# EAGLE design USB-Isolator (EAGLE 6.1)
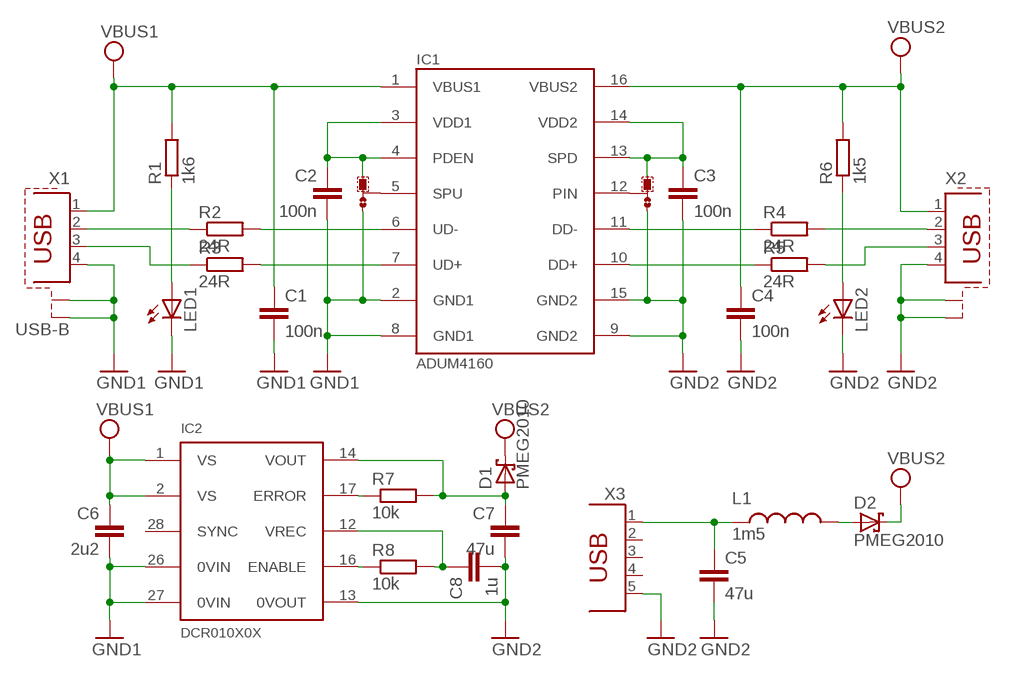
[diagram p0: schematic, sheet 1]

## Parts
C1  100n  C-EUC1206  [C1206]
C2  100n  C-EUC1206  [C1206]
C3  100n  C-EUC1206  [C1206]
C4  100n  C-EUC1206  [C1206]
C5  47u  C-EUC1210  [C1210]
C6  2u2  C-EUC1206  [C1206]
C7  47u  C-EUC1210  [C1210]
C8  1u  C-EUC1206  [C1206]
D1  PMEG2010  [SOD523]
D2  PMEG2010  [SOD523]
IC1  ADUM4160  ADUM4160BRWZ  [SOIC16W]
IC2  DCR010X0X  [SO28-3/12]
JMP1  0R-JUMPA  [A0R-JMP]
JMP2  0R-JUMPA  [A0R-JMP]
L1  1m5  L-1206  [L1206]
LED1  LED3MM  [LED3MM]
LED2  LED3MM  [LED3MM]
R1  1k6  R-EU_M1206  [M1206]
R2  24R  R-EU_M1206  [M1206]
R3  24R  R-EU_M1206  [M1206]
R4  24R  R-EU_M1206  [M1206]
R5  24R  R-EU_M1206  [M1206]
R6  1k5  R-EU_M1206  [M1206]
R7  10k  R-EU_M1206  [M1206]
R8  10k  R-EU_M1206  [M1206]
X1  USB-B  [USB-B]
X2  USB-A-SMD  [USB-A-SMD]
X3  USB-MINI-B-SMD  [USB-MINI-B-SMD]

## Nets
0V: C3.2 C4.2 C5.2 C7.2 C8.2 IC1.9(GND2) IC1.15(GND2) IC2.13(0VOUT) JMP2.3 LED2.K(C) X2.4 X2.P$1(S1) X2.P$2(S2) X3.5 ; supply symbol labelled GND2
GND: C1.2 C2.2 C6.2 IC1.2(GND1) IC1.8(GND1) IC2.26(0VIN) IC2.27(0VIN) JMP1.3 LED1.K(C) X1.4 X1.S1 X1.S2 ; supply symbol labelled GND1
N$1: R2.1 X1.2
N$2: IC1.6(UD-) R2.2
N$3: R3.1 X1.3
N$4: IC1.7(UD+) R3.2
N$5: LED1.A R1.1
N$6: IC1.11(DD-) R4.1
N$7: IC1.10(DD+) R5.1
N$8: R5.2 X2.3
N$9: R4.2 X2.2
N$10: LED2.A R6.1
N$11: IC1.5(SPU) JMP1.2
N$12: IC1.12(PIN) JMP2.2
N$13: C5.1 L1.1 X3.1
N$14: IC2.17(ERROR) R7.1
N$15: IC2.16(ENABLE) R8.1
N$16: C8.1 IC2.12(VREC) R8.2
N$17: D2.A L1.2
N$18: C7.1 D1.A IC2.14(VOUT) R7.2
VBUS1: C1.1 C6.1 IC1.1(VBUS1) IC2.1(VS) IC2.2(VS) R1.2 X1.1
VBUS2: C4.1 D1.C D2.C IC1.16(VBUS2) R6.2 X2.1
VDD1: C2.1 IC1.3(VDD1) IC1.4(PDEN) JMP1.1
VDD2: C3.1 IC1.13(SPD) IC1.14(VDD2) JMP2.1
Unconnected: IC2.28(SYNC) X3.2 X3.3 X3.4

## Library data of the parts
C1-C8 = rcl:C-EU: CAPACITOR, European symbol
D1 D2 = USB-Isolator:PMEG2010
IC1 = USB-Isolator:ADUM4160BRWZ
IC2 = USB-Isolator:DCR010X0X: DC/DC Converter DC010505 RS NR 5412.5189.00
JMP1 JMP2 = jump-0r-smd:0R-JUMP: SMD 0R 0805 Jumper
L1 = USB-Isolator:L-1206
LED1 LED2 = led:LED: LED
R1-R8 = rcl:R-EU_: RESISTOR, European symbol
X1 = USB-Isolator:USB-B; OC_FARNELL: unknown; OC_NEWARK: unknown
X2 = USB-Isolator:USB-A-SMD
X3 = USB-Isolator:USB-MINI-B-SMD

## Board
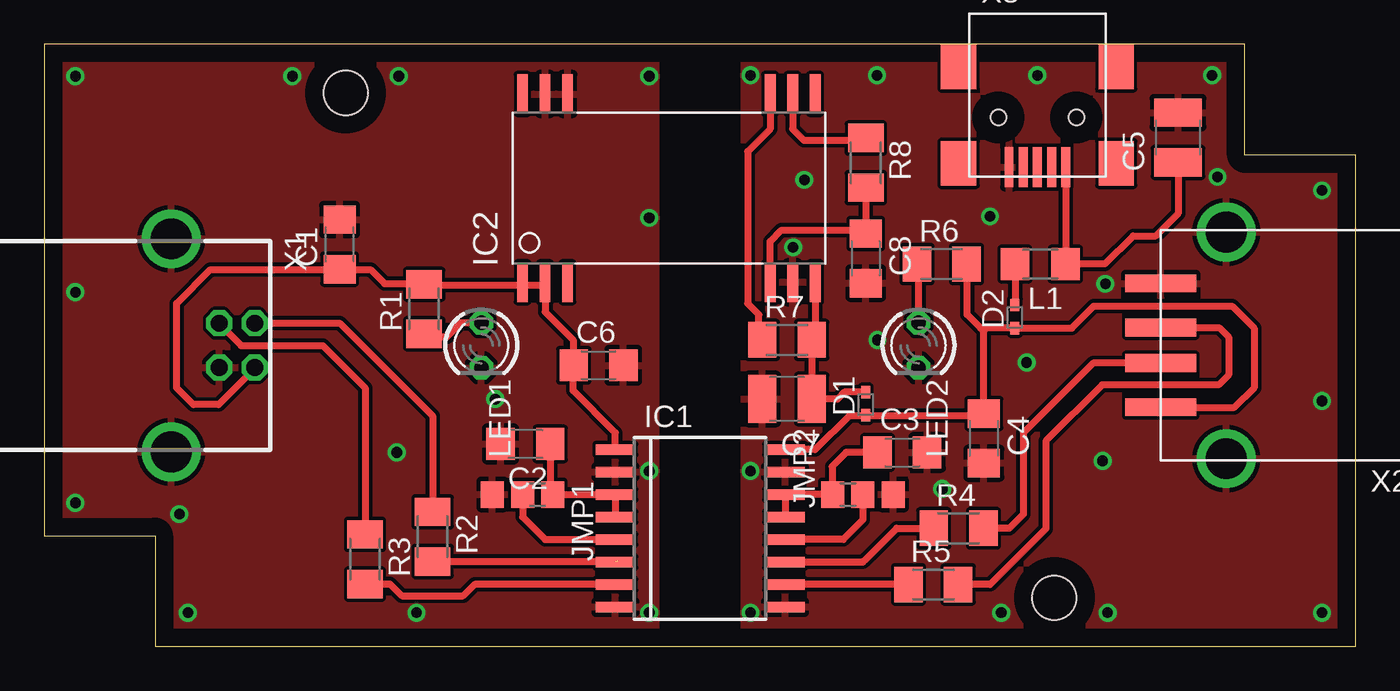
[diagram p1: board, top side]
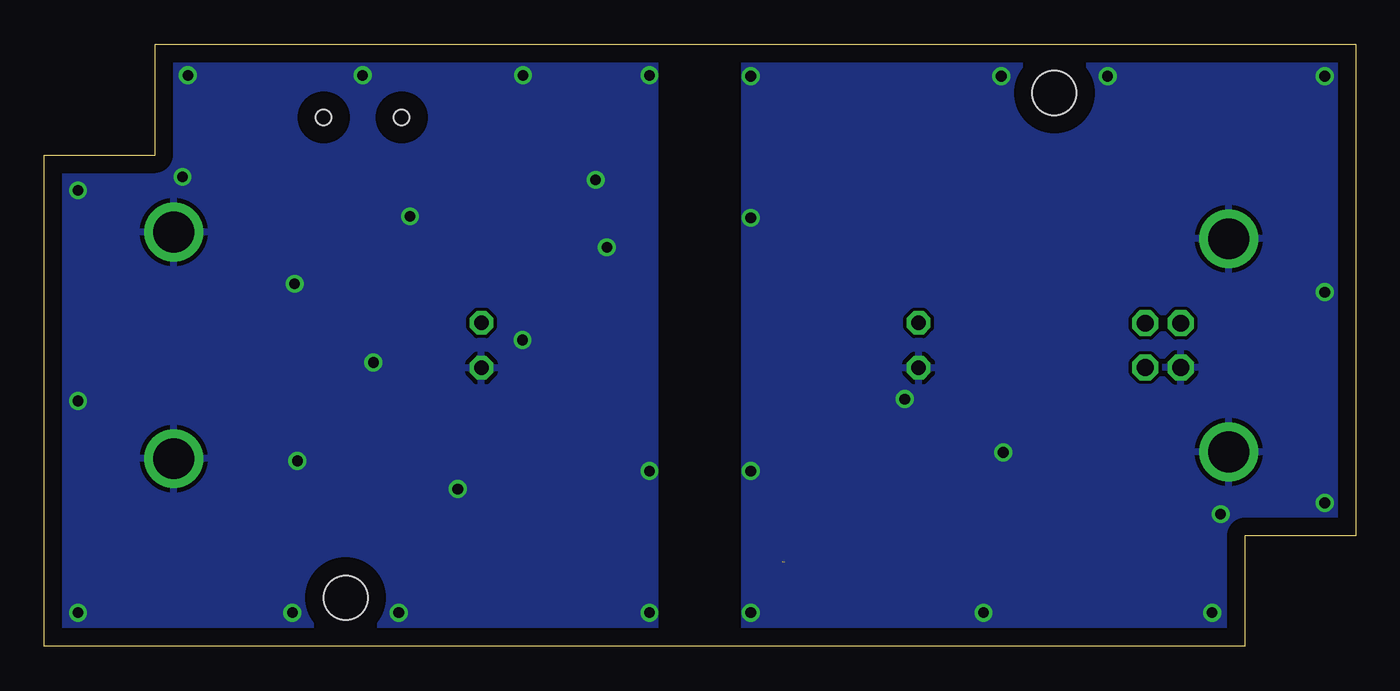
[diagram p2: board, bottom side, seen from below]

Size 74 x 34 mm. Coordinates in mm from the lower left corner, seen from the top.
Outline: 0,34 0,6.25 6.25,6.25 6.25,0 74,0 74,27.75 67.75,27.75 67.75,34 0,34
Copper layers (1*16): Top 0.035mm / dielectric 1.5mm / Bottom 0.035mm
Design rules: minimum track width 10mil, minimum drill 24mil, track to track 8mil, track to pad 8mil, pad to pad 8mil, via to via 8mil, smd to smd 8mil, copper to edge 40mil, drill to drill 8mil, minimum pad ring 10mil, minimum via ring 8mil, stop-mask expansion 4mil, vias tented up to drill 0mil, thermal gap 10mil
Holes 2.5 mm at 17,31.25 57,2.75

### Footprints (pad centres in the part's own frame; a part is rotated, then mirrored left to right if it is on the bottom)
C1206 = smd 1.6 x 1.8: 1 -1.4,0; 2 1.4,0
C1210 = smd 1.6 x 2.7: 1 -1.4,0; 2 1.4,0
SOD523 = smd 0.7 x 0.5: A 0.7,0; C -0.6,0
SOIC16W = smd 0.6 x 2.2: 1 -4.445,-4.775; 2 -3.175,-4.775; 3 -1.905,-4.775; 4 -0.635,-4.775; 5 0.635,-4.775; 6 1.905,-4.775; 7 3.175,-4.775; 8 4.445,-4.775; 9 4.445,4.8; 10 3.175,4.8; 11 1.905,4.8; 12 0.635,4.8; 13 -0.635,4.8; 14 -1.905,4.8; 15 -3.175,4.8; 16 -4.445,4.8
SO28-3/12 = smd 0.61 x 2.21: 1 -8.255,-5.315; 2 -6.985,-5.315; 3 -5.715,-5.315; 12 5.715,-5.315; 13 6.985,-5.315; 14 8.255,-5.315; 15 8.255,5.315; 16 6.985,5.315; 17 5.715,5.315; 26 -5.715,5.315; 27 -6.985,5.315; 28 -8.255,5.315
A0R-JMP = smd 1.5 x 1.3: 1 0,1.7; 2 0,0; 3 0,-1.7
L1206 = smd 1.6 x 1.803: 1 -1.422,0; 2 1.422,0
LED3MM = drill 0.813 octagon: A -1.27,0; K 1.27,0
M1206 = smd 1.6 x 2: 1 -1.4,0; 2 1.4,0
USB-B = drill 0.95 octagon: 1 1.25,4.71; 2 -1.25,4.71; 3 -1.25,2.71; 4 1.25,2.71 | drill 2.3 pad 2.9: S1 -6.02,0; S2 6.02,0
USB-A-SMD = smd 4 x 1: 1 0,3.5; 2 0,1; 3 0,-1; 4 0,-3.5 | drill 2.3 pad 2.9: P$1 -3.7,6.4; P$2 -3.7,-6.4
USB-MINI-B-SMD = smd 0.5 x 2.25: 1 -1.6,3.57; 2 -0.8,3.57; 3 0,3.57; 4 0.8,3.57; 5 1.6,3.57 | smd 2 x 2.5: C1 -4.45,3.37; C2 -4.45,-2.08; C3 4.45,-2.08; C4 4.45,3.37 | hole 0.9: 2.2,0.77; -2.2,0.77

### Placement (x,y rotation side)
C1  16.67,22.7 90 top
C2  27.15,11.43 180 top
C3  48.42,10.95 0 top
C4  53.02,11.75 270 top
C5  63.98,28.73 90 top
C6  31.27,15.88 0 top
C7  41.91,13.97 180 top
C8  46.35,21.91 270 top
D1  46.35,13.65 90 top
D2  54.77,18.57 90 top
IC1  37,6.67 270 top
IC2  35.24,25.88 0 top
JMP1  26.99,8.57 270 top
JMP2  46.2,8.57 90 top
L1  56.2,21.59 180 top
LED1  24.66,17 270 top
LED2  49.33,17 270 top
R1  21.43,19.05 90 top
R2  21.91,6.19 270 top
R3  18.1,4.92 270 top
R4  51.59,6.67 0 top
R5  50.16,3.49 0 top
R6  50.64,21.59 0 top
R7  41.91,17.3 0 top
R8  46.35,27.3 270 top
X1  7.16,17 270 top
X2  63,17 180 top
X3  56.04,30.64 180 top

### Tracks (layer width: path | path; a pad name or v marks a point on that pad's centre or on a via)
0V  (via drill 0.6)
  other vias: 56.04,32.25 65.9,32.25 72.1,25.75 66.2,26.51 72.1,1.9 46.99,32.25 39.85,32.25 39.85,9.9 39.85,1.9 72.1,13.86 60,1.9 54,1.9 50.67,8.88 53.37,24.28 47.02,17.3 55.43,16.03 59.72,10.47 42.26,22.54 59.88,20.47 42.89,26.35
  pour Top: 39.5,34 74,34 74,0 39.5,0
  pour Bottom: 39.53,34 74.03,34 74.03,0 39.53,0
GND  (via drill 0.6)
  other vias: 1.75,32.2 1.75,8.1 8.1,1.9 7.62,7.46 14,32.2 20,32.2 34.13,32.2 34.13,9.9 34.13,1.9 34.13,24.2 21,1.9 19.89,10.95 25.45,13.96 1.75,20
  pour Top: 0,34 34.5,34 34.5,0 0,0
  pour Bottom: 0,34 34.5,34 34.5,0 0,0
N$1
  Top 0.406: X1.2 14.88,18.26 16.67,18.26 21.91,13.02 R2.1
N$2  (1 unrouted)
  Top 0.406: R2.2 32.36,4.79 32.38,4.76
N$3
  Top 0.406: R3.1 18.1,14.61 15.72,16.99 11.11,16.99 9.87,18.23 X1.3
N$4
  Top 0.406: R3.2 19.5,3.52 20.16,2.86 23.65,2.86 24.29,3.49 IC1.7
N$5
  Top 0.406: LED1.A 23.51,18.27 22.7,17.46 20.98,17.46 R1.1
N$6
  Top 0.406: R4.1 48.1,6.67 47.15,5.71 46.35,4.92 46.2,4.76 IC1.11
N$7
  Top 0.406: R5.1 IC1.10
N$8
  Top 0.406: 51.91,3.49 53.37,3.49 56.52,6.64 56.52,11.59 59.69,14.76 66.26,14.76 66.83,15.34 66.83,17.46 66.3,18 X2.3 | 51.91,3.49 51.75,3.65 | 51.91,3.33 51.75,3.49 R5.2 51.91,3.49
N$9
  Top 0.406: X2.2 59.18,16 55.24,12.06 55.24,7.46 54.45,6.67 R4.2
N$10
  Top 0.406: LED2.A 49.33,21.66 R6.1
N$11
  Top 0.406: JMP1.2 26.99,7.3 28.26,6.03 IC1.5
N$12
  Top 0.406: JMP2.2 46.2,7.14 45.09,6.03 IC1.12
N$13
  Top 0.406: X3.1 57.64,21.74 57.71,21.67 | 57.71,21.67 57.78,21.59 | 57.71,21.67 L1.1 59.85,21.59 61.44,23.18 62.71,23.18 63.98,24.45 C5.1
N$14
  Top 0.406: IC2.17 40.96,29.21 39.69,27.94 39.69,19.37 40.32,18.73 40.32,17.02 R7.1
N$15
  Top 0.406: IC2.16 42.23,29.21 42.86,28.57 46.35,28.57 R8.1
N$16
  Top 0.406: R8.2 C8.1 46.17,23.5 41.59,23.5 40.96,22.86 IC2.12
N$17
  Top 0.406: L1.2 54.78,19.37 | 54.78,19.37 54.77,19.37 | 54.78,19.37 D2.A
N$18
  Top 0.406: IC2.14 43.5,17.02 R7.2 | R7.2 43.31,16.96 43.34,16.99 | R7.2 43.31,14.26 | 43.31,14.26 43.18,14.13 C7.1 | 43.31,14.26 C7.1 | C7.1 43.18,13.97 | D1.A 45.15,14.35 44.77,13.97 C7.1
VBUS1
  Top 0.406: 16.7,21.27 9.37,21.27 7.46,19.37 7.46,14.61 8.41,13.65 9.84,13.65 11.87,15.68 X1.1 | 16.7,21.27 18.41,21.27 19.21,20.48 21.46,20.48 | IC1.1 32.23,12.07 29.84,14.45 29.84,15.74 C6.1 | 29.84,16.19 29.84,16.03 29.71,16.16 C6.1 | 29.69,16.22 C6.1 | 16.7,21.27 C1.1 | 21.59,20.48 21.46,20.48 | 21.46,20.48 R1.2 21.4,20.48 20.64,20.48 20.71,20.4 27.15,20.4 | IC2.2 28.26,20.48 28.18,20.4 | 29.53,15.88 29.69,15.72 | 29.69,15.72 29.69,15.56 | 29.69,15.72 29.69,15.85 C6.1 | 27.15,20.4 28.18,20.4 | IC2.1 27.15,20.4 | 28.18,20.4 28.18,20.24 28.26,20.16 28.26,18.89 29.84,17.3 29.84,15.9 C6.1
VBUS2
  Top 0.406: 41.75,11.11 IC1.16 43.5,11.11 45.44,13.05 46.32,13.05 46.35,13.02 D1.C 52.93,13.05 C4.1 53.02,17.78 52.83,17.97 | 52.83,17.97 D2.C 57.98,17.97 59.21,19.21 67.02,19.21 68.26,17.97 68.26,14.61 67.16,13.5 X2.1 | 52.83,17.97 52.07,18.73 52.07,21.72 R6.2
VDD1
  Top 0.406: 32.38,7.3 32.23,7.46 IC1.3 JMP1.1 | 32.38,7.3 33.02,7.3 | 32.38,7.3 IC1.4 | JMP1.1 28.89,8.57 | JMP1.1 28.57,8.57 | 28.57,8.57 28.26,8.57 | C2.1 28.55,8.6 28.57,8.57
VDD2
  Top 0.406: IC1.13 IC1.14 JMP2.1 44.61,8.57 44.45,8.73 44.45,10.16 45.24,10.95 C3.1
